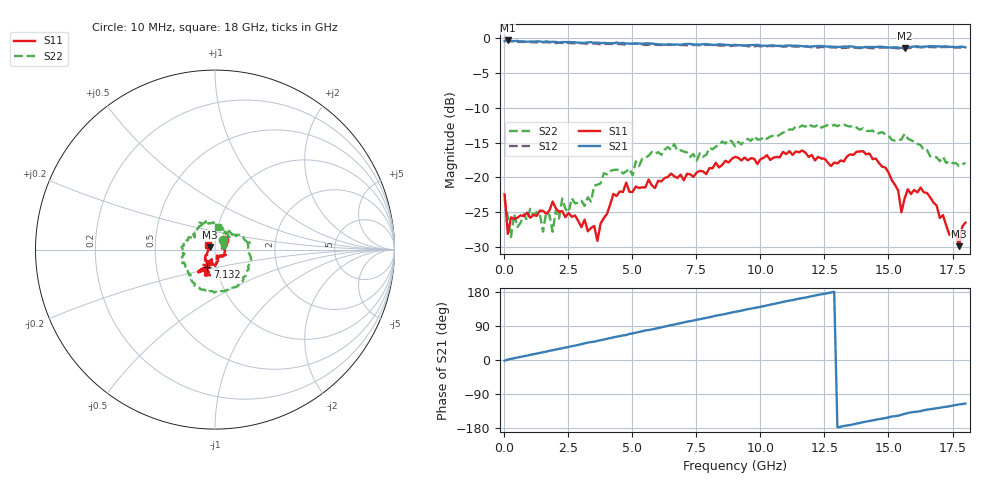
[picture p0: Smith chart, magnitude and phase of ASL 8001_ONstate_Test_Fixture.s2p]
!ASL 8001 Wideband SPST Switch
!ON State Test Fixture S-parameter data from 10MHz-18 GHz
!Agilent Technologies,E8363B,MY43030569,A.06.01.05
!Agilent E8363B: A.06.01.05
!Date: Wednesday, November 15, 2006 16:46:40
!Correction: S11(Full 2 Port(1,2)) S21(Full 2 Port(1,2)) S12(Full 2 Port(1,2)) S22(Full 2 Port(1,2))
!S2P File: Measurements: S11, S21, S12, S22:
# Hz S  dB  R 50
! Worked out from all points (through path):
!   145 points, 10 MHz to 18 GHz, reference 50 ohm
!   highest |S21| = -0.34 dB at 134.9 MHz (marker M1); lowest = -1.5 dB at 15.63 GHz (marker M2)
!   lowest |S11| = -29.9 dB at 17.75 GHz (marker M3), VSWR 1.07, Z = 47.2 + j1.33 ohm
!   |S11| at or under -10 dB: start of sweep to end of sweep
!   |S22| runs from -28.5 to -12.3 dB; largest |S21 - S12| = 0.045
!   S11 on the Smith chart (normalised r, x): 10 MHz: 1.10, +0.12; 7.132 GHz: 0.90, -0.18; 18 GHz: 0.92, +0.05
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1e7  -22.43 46.7  -0.42 -1.8  -0.44 -4.5  -23.12 49.9
1.3495e8  -28.11 10.6  -0.34 1.3  -0.46 1.1  -25.68 20.1
2.599e8  -25.74 10.2  -0.42 3.1  -0.46 3.0  -28.55 20.4
3.8485e8  -25.96 6.0  -0.44 4.7  -0.49 4.7  -25.22 28.8
5.098e8  -25.79 12.8  -0.40 6.7  -0.55 6.4  -27.12 23.7
1.0096e9  -25.78 11.2  -0.51 13.6  -0.59 13.2  -24.51 28.2
1.88425e9  -23.47 -25.7  -0.55 25.7  -0.69 25.6  -27.79 16.8
2.2591e9  -24.84 -41.4  -0.57 31.2  -0.70 30.9  -23.05 18.9
3.0088e9  -27.13 -47.0  -0.68 41.7  -0.75 41.5  -23.34 27.5
3.63355e9  -29.10 -69.4  -0.65 50.4  -0.83 50.4  -21.05 34.3
4.2583e9  -22.35 -84.8  -0.75 59.9  -0.84 59.3  -18.93 47.5
6.0076e9  -20.47 -117.6  -0.91 84.3  -0.98 84.2  -16.38 104.4
7.13215e9  -19.48 -114.0  -0.86 101.2  -1.03 100.4  -16.41 131.3
9.0064e9  -17.05 -123.3  -0.96 127.2  -1.08 127.3  -15.54 -177.4
1.20052e10  -16.78 -124.8  -1.19 168.4  -1.34 168.3  -12.63 -98.5
1.40044e10  -16.23 -111.2  -1.34 -164.1  -1.43 -164.5  -12.95 -40.5
1.5004e10  -19.31 -114.2  -1.35 -151.4  -1.40 -151.4  -14.03 -9.6
1.55038e10  -25.01 -108.3  -1.43 -144.5  -1.56 -144.9  -14.58 11.3
1.562875e10  -23.03 -104.0  -1.46 -142.2  -1.58 -142.2  -13.74 11.7
1.65034e10  -22.24 -137.5  -1.22 -131.1  -1.29 -131.4  -16.06 31.5
1.77529e10  -29.87 154.0  -1.26 -117.1  -1.37 -117.6  -18.35 68.6
1.80028e10  -26.48 144.4  -1.33 -114.8  -1.44 -115.3  -17.89 82.1
